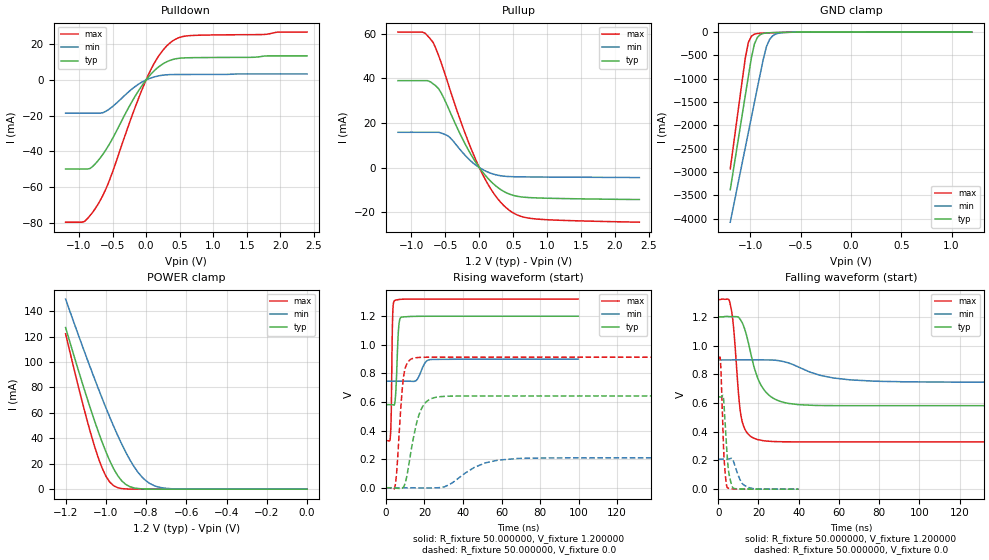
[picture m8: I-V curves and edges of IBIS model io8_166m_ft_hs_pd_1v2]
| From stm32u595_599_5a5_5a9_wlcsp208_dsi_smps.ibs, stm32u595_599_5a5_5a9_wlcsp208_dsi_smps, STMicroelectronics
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|   Model io8_166m_ft_hs_pd_1v2
[Model]  io8_166m_ft_hs_pd_1v2
Model_type I/O
Polarity   Non-Inverting
Enable   Active-Low
Vinl =   0.360000V
Vinh =   0.840000V
Vmeas =  0.600000V
Cref =   50.000000pF
Rref =   100.000000M
Vref =   0.0V
C_comp   3.151500pF   3.086800pF   3.197700pF
[Temperature Range]   25.000000   0.140000k   -40.000000
[Pullup Reference]   1.200000V   0.900000V   1.320000V
[Pulldown Reference]   0.0V   0.0V   0.0V
[POWER Clamp Reference]   1.200000V   0.900000V   1.320000V
[GND Clamp Reference]   0.0V   0.0V   0.0V
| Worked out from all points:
|   slope of the pulldown table from 0 to 0.18 V, typ, clamps not added: 25.4 ohm
|   slope of the pullup table from 0 to 0.18 V, typ, clamps not added: 27.8 ohm
|   GND clamp passes 1 mA (typ) near -0.51 V on its own axis
|   POWER clamp passes 1 mA (typ) near -0.86 V on its own axis
|   rising waveform, R_fixture 50.000000, V_fixture 1.200000: 20-80 % time 1.12ns typ, 3.04ns min, 582ps max; typ from 0.581 V to 1.2 V
|   rising waveform, R_fixture 50.000000, V_fixture 0.0: 20-80 % time 5.79ns typ, 15.1ns min, 2.79ns max; typ from 0 V to 0.642 V
|   falling waveform, R_fixture 50.000000, V_fixture 1.200000: 20-80 % time 8.14ns typ, 19.6ns min, 3.49ns max; typ from 1.2 V to 0.581 V
|   falling waveform, R_fixture 50.000000, V_fixture 0.0: 20-80 % time 1.93ns typ, 3.59ns min, 1.45ns max; typ from 0.642 V to 0 V
[Pulldown]
|Voltage   I(typ)   I(min)   I(max)
-1.2V     -49.86mA   -18.57mA   -79.56mA
-920mV    -49.86mA   -18.57mA   -79.19mA
-840mV    -49.6mA    -18.57mA   -76.08mA
-720mV    -45.32mA   -18.57mA   -69.74mA
-560mV    -36.71mA   -16.58mA   -57.44mA
-200mV    -11.43mA   -4.74mA    -19.03mA
0V        -10fA      -500fA     0A
160mV     6.477mA    2.075mA    11.78mA
360mV     10.99mA    2.99mA     20.81mA
480mV     12.07mA    3.054mA    23.53mA
640mV     12.43mA    3.075mA    24.76mA
2.4V      13.46mA    3.37mA     26.78mA
[Pullup]
|Voltage   I(typ)   I(min)   I(max)
-1.2V     38.94mA    15.8mA     60.7mA
-840mV    38.94mA    15.8mA     60.7mA
-680mV    37.51mA    15.8mA     56.01mA
-600mV    35.31mA    15.8mA     50.19mA
-440mV    25.54mA    13.66mA    35.67mA
-240mV    12.39mA    6.512mA    17.85mA
-40mV     1.772mA    818.2uA    2.67mA
200mV     -7.072mA   -2.851mA   -11mA
440mV     -11.84mA   -4.03mA    -19.1mA
600mV     -13.07mA   -4.154mA   -21.71mA
840mV     -13.59mA   -4.223mA   -23.04mA
2.36V     -14.3mA    -4.5mA     -24.47mA
[GND_clamp]
|Voltage   I(typ)   I(min)   I(max)
-1.2V     -3.379A    -4.076A    -2.932A
-1.05V    -1.35A     -2.47A     -550.7mA
-1.02V    -947.8mA   -2.15A     -221.5mA
-990mV    -552.4mA   -1.829A    -88.45mA
-960mV    -255.3mA   -1.51A     -44.89mA
-930mV    -111.8mA   -1.191A    -30.7mA
-870mV    -28.37mA   -564.6mA   -21.36mA
-840mV    -18.66mA   -309.5mA   -18.51mA
-810mV    -14.08mA   -161.6mA   -15.94mA
-780mV    -11.38mA   -83.33mA   -13.55mA
-600mV    -3.02mA    -4.329mA   -3.104mA
1.2V      30.28uA    18.17uA    37.27uA
[POWER_clamp]
|Voltage   I(typ)   I(min)   I(max)
-1.2V     127mA      149.4mA    122.2mA
-1.12V    84.97mA    114mA      70.27mA
-1.06V    55.51mA    88.42mA    35.67mA
-1.02V    37.63mA    72.04mA    17.17mA
-1V       29.51mA    64.13mA    10.3mA
-960mV    15.69mA    48.99mA    2.571mA
-900mV    3.624mA    28.77mA    182.8uA
-840mV    490.7uA    13.24mA    11.35uA
-800mV    116.8uA    6.532mA    1.77uA
-740mV    13.2uA     1.724mA    109.1nA
-620mV    167.4nA    79.36uA    0A
0V        0A         17.87nA    0A
[Ramp]
| variable   typ   min   max
dV/dt_r  0.38527/5.78263n   0.12539/15.12854n   0.54788/2.78067n
dV/dt_f  0.37097/8.13487n   92.64000m/19.56169n 0.59419/3.47998n
R_load = 50.000000
[Rising Waveform]
R_fixture= 50.000000
V_fixture= 1.200000
V_fixture_min= 0.900000
V_fixture_max= 1.320000
|time   V(typ)   V(min)   V(max)
0s        581.2mV    745.1mV    329.2mV
2.402ns   581.3mV    745.1mV    368.1mV
2.803ns   581.3mV    745.1mV    528.3mV
3.203ns   580.9mV    745.1mV    974.6mV
3.604ns   579.7mV    745.1mV    1.234V
4.404ns   579.8mV    745.1mV    1.307V
6.607ns   1.115V     745.1mV    1.316V
7.808ns   1.191V     745.1mV    1.318V
23.02ns   1.199V     896.1mV    1.319V
99.7ns    1.2V       899.5mV    1.319V
[Rising Waveform]
R_fixture= 50.000000
V_fixture= 0.0
V_fixture_min= 0.0
V_fixture_max= 0.0
|time   V(typ)   V(min)   V(max)
0s        1.413uV    1.123uV    1.262uV
4.805ns   -1.542mV   770.6nV    12.85mV
5.606ns   -3.324mV   635.9nV    108.6mV
9.209ns   6.524mV    -358.8nV   778.1mV
11.21ns   105.2mV    6.305uV    875.3mV
14.01ns   330.2mV    38.85uV    904.9mV
19.22ns   570.8mV    -1.423mV   912.2mV
28.03ns   636.7mV    1.435mV    913mV
58.06ns   642mV      192.9mV    913.1mV
199.4ns   642.1mV    209.1mV    913.1mV
[Falling Waveform]
R_fixture= 50.000000
V_fixture= 1.200000
V_fixture_min= 0.900000
V_fixture_max= 1.320000
|time   V(typ)   V(min)   V(max)
0s        1.2V       899.5mV    1.319V
5.606ns   1.201V     899.4mV    1.31V
7.207ns   1.201V     899.8mV    1.185V
10.41ns   1.193V     900.6mV    614.4mV
11.61ns   1.167V     900.5mV    490.6mV
19.22ns   790.3mV    899.9mV    346.9mV
26.43ns   641.5mV    899.2mV    332.3mV
40.04ns   588.1mV    849.3mV    329.3mV
77.68ns   581.2mV    751.6mV    329.2mV
199.4ns   581.2mV    745.1mV    329.2mV
[Falling Waveform]
R_fixture= 50.000000
V_fixture= 0.0
V_fixture_min= 0.0
V_fixture_max= 0.0
|time   V(typ)   V(min)   V(max)
0s        642.1mV    209.1mV    913.1mV
1.201ns   642mV      209.1mV    874.9mV
2.563ns   641.8mV    209.1mV    327.2mV
3.443ns   463.2mV    209mV      118.1mV
4.484ns   230.8mV    208.8mV    12.13mV
5.606ns   90.11mV    211.2mV    4.551mV
7.768ns   4.908mV    187.6mV    1.226mV
11.61ns   1.202mV    46.29mV    349.1uV
15.38ns   575.4uV    10.79mV    142.7uV
39.88ns   1.413uV    1.123uV    1.262uV
